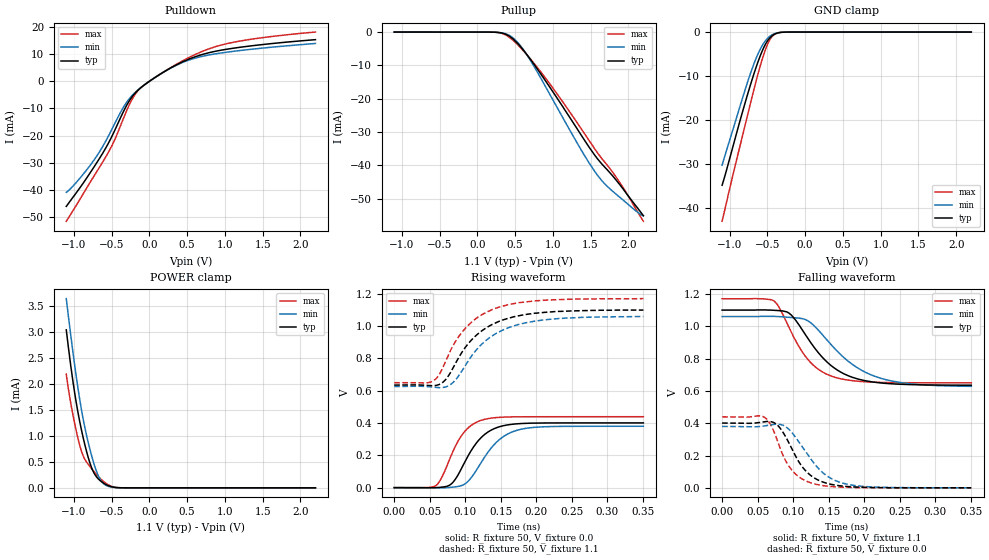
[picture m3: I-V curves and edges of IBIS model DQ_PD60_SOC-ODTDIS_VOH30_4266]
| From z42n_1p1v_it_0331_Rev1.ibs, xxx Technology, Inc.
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| DQ_PD60_SOC-ODTDIS_VOH30_4266
| (60 Ohm Pulldown, SOC ODT disabled setting, VOH=VDDQ/3.0 cal. point, 3200-4266Mbps)
[Model]   DQ_PD60_SOC-ODTDIS_VOH30_4266
Model_type   I/O
Vinl = 123.333mV
Vinh = 243.333mV
Vmeas = 183.333mV
Vref = 0.0mV
Cref = 0.0pF
|   typ   min   max
|C_comp   0.834pF   0.784pF   0.884pF
C_comp_pullup   0.4170pF   0.3920pF   0.4420pF
C_comp_pulldown   0.4170pF   0.3920pF   0.4420pF
| Note: C_comp changes when the ODT circuit is enabled.
[Model Spec]
| Input threshold voltage corners
Vinl   0.1233V   0.1167V   0.1350V
Vinh   0.2433V   0.2367V   0.2550V
| Measurement voltage corners
Vmeas   0.1833V   0.1767V   0.1950V
| Timing spec test load voltage corners
Vref   0.0000V   0.0000V   0.0000V
| Dynamic Overshoot Parameters from LPDDR4 Specification
D_overshoot_ampl_h   0.30   NA   NA
D_overshoot_ampl_l   0.30   NA   NA
D_overshoot_area_h   0.1n   NA   NA
D_overshoot_area_l   0.1n   NA   NA
[Voltage Range]   1.1000V   1.0600V   1.1700V
[Pullup Reference]   1.1000V   1.0600V   1.1700V
| Junction Temperature (Ambient temp is 35C typ 95C min -40C max)
[Temperature Range]   50.0   110.0   -40.0
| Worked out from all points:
|   slope of the pulldown table from 0 to 0.165 V, typ, clamps not added: 54.8 ohm
|   slope of the pullup table from 0 to 0.165 V, typ, clamps not added: 13 kohm
|   GND clamp passes 1 mA (typ) near -0.45 V on its own axis
|   POWER clamp passes 1 mA (typ) near -0.88 V on its own axis
|   rising waveform, R_fixture 50, V_fixture 0.0: 20-80 % time 35ps typ, 39ps min, 30.3ps max; typ from 0.001 V to 0.401 V
|   falling waveform, R_fixture 50, V_fixture 1.1: 20-80 % time 54ps typ, 66.1ps min, 43.5ps max; typ from 1.1 V to 0.635 V
|   rising waveform, R_fixture 50, V_fixture 1.1: 20-80 % time 55.1ps typ, 57.5ps min, 52.4ps max; typ from 0.635 V to 1.1 V
|   falling waveform, R_fixture 50, V_fixture 0.0: 20-80 % time 34.8ps typ, 42ps min, 30.2ps max; typ from 0.401 V to 0.001 V
[Pulldown]
|   Voltage   I(typ)   I(min)   I(max)
-1.1V     -46.14mA   -40.94mA   -51.62mA
-918.5mV  -39.24mA   -35.7mA    -43.49mA
-710.6mV  -30.65mA   -28.16mA   -33.97mA
-492.8mV  -20.14mA   -17.52mA   -23.58mA
-357.5mV  -12.02mA   -10.26mA   -14.71mA
-265.1mV  -7.208mA   -6.415mA   -8.684mA
-172.7mV  -3.892mA   -3.712mA   -4.234mA
-60.5mV   -1.24mA    -1.226mA   -1.224mA
411.4mV   6.776mA    6.592mA    7.095mA
893.2mV   11.15mA    10.18mA    12.89mA
1.365V    13.11mA    11.84mA    15.56mA
2.2V      15.34mA    13.95mA    18.15mA
[GND Clamp]
|   Voltage   I(typ)   I(min)   I(max)
-1.1V     -34.74mA   -30.21mA   -42.91mA
-1.047V   -31.66mA   -27.15mA   -39.02mA
-941.6mV  -25.02mA   -21.26mA   -31.32mA
-789.8mV  -15.72mA   -12.78mA   -20.72mA
-667.7mV  -8.907mA   -6.722mA   -12.29mA
-595.1mV  -5.399mA   -3.899mA   -7.688mA
-522.5mV  -2.666mA   -1.905mA   -3.811mA
-469.7mV  -1.359mA   -987.8uA   -1.786mA
-413.6mV  -563.7uA   -416.4uA   -619.9uA
-344.3mV  -144.1uA   -109.8uA   -124.4uA
-238.7mV  -9.035uA   -8.519uA   -5.04uA
2.2V      0A         0A         0A
[Pullup]
|   Voltage   I(typ)   I(min)   I(max)
-1.1V     6.275uA    9.671uA    2.829uA
229.9mV   -45.12uA   -45.81uA   -46.58uA
338.8mV   -360.2uA   -298.3uA   -496uA
434.5mV   -1.385mA   -1.132mA   -1.75mA
553.3mV   -3.878mA   -3.573mA   -4.208mA
691.9mV   -7.808mA   -8.045mA   -7.726mA
1.009V    -18.16mA   -20.62mA   -17.03mA
1.378V    -30.95mA   -35.41mA   -29.04mA
1.589V    -37.92mA   -42.84mA   -36.13mA
1.702V    -40.84mA   -45.82mA   -39.37mA
1.89V     -45.83mA   -49.59mA   -45.19mA
2.2V      -55.05mA   -55.17mA   -56.74mA
[POWER Clamp]
|   Voltage   I(typ)   I(min)   I(max)
-1.1V     3.033mA    3.633mA    2.184mA
-1.041V   2.345mA    2.929mA    1.625mA
-984.5mV  1.782mA    2.31mA     1.205mA
-911.9mV  1.201mA    1.61mA     764.7uA
-855.8mV  837.7uA    1.171mA    552.1uA
-779.9mV  447.9uA    701.4uA    396.3uA
-710.6mV  232.3uA    359.1uA    273.1uA
-657.8mV  146.8uA    178.8uA    190.7uA
-595.1mV  80.76uA    68.28uA    109.2uA
-482.9mV  15.73uA    9.557uA    19.51uA
-360.8mV  1.018uA    768.5nA    796.1nA
2.2V      0A         0A         0A
[Ramp]
|   typ   min   max
| 20% - 80%
dV/dt_r   240.24m/34.97p   227.79m/39.04p   263.30m/30.33p
dV/dt_f   278.79m/54.03p   259.05m/66.11p   312.07m/43.50p
| 25% - 75%
|dV/dt_r   200.20m/27.85p   189.82m/31.09p   219.41m/24.09p
|dV/dt_f   232.33m/43.03p   215.87m/52.69p   260.06m/34.62p
R_load = 50
[Rising Waveform]
R_fixture = 50
V_fixture = 0.0
|   Time   V(typ)   V(min)   V(max)
0s        701.6uV    613.5uV    508.4uV
58ps      514.8uV    -95.55uV   11.58mV
66ps      3.219mV    -535uV     55.51mV
78ps      15.84mV    1.701mV    175.5mV
87ps      58.39mV    5.992mV    264.1mV
99ps      155.2mV    21.91mV    346.3mV
125ps     320.7mV    173.6mV    420.4mV
150ps     379.7mV    304.4mV    436.1mV
179ps     397.3mV    362.2mV    439mV
351ps     401.1mV    380.3mV    439.3mV
[Falling Waveform]
R_fixture   = 50
V_fixture   = 1.1
V_fixture_min = 1.06
V_fixture_max = 1.17
|   Time   V(typ)   V(min)   V(max)
0s        1.1V       1.06V      1.17V
73ps      1.099V     1.061V     1.157V
94ps      1.082V     1.055V     995mV
118ps     943.4mV    1.04V      810mV
135ps     839.3mV    978.7mV    735.6mV
155ps     751.6mV    879mV      689.9mV
187ps     679.1mV    753.1mV    661.6mV
224ps     649mV      677.5mV    652.7mV
271ps     638.3mV    641.5mV    650.4mV
351ps     635.3mV    628.2mV    649.9mV
[Rising Waveform]
R_fixture   = 50
V_fixture   = 1.1
V_fixture_min = 1.06
V_fixture_max = 1.17
|   Time   V(typ)   V(min)   V(max)
0s        635mV      626.1mV    649.8mV
54ps      631.1mV    622.7mV    658.9mV
64ps      640mV      619.2mV    704.7mV
77ps      696.3mV    631.8mV    828.3mV
91ps      806.6mV    693.5mV    936mV
109ps     914.8mV    814.9mV    1.024V
127ps     981.8mV    902.8mV    1.079V
148ps     1.03V      965mV      1.118V
210ps     1.084V     1.038V     1.16V
351ps     1.099V     1.059V     1.17V
[Falling Waveform]
R_fixture = 50
V_fixture = 0.0
|   Time   V(typ)   V(min)   V(max)
0s        401.2mV    380.4mV    439.4mV
57ps      408mV      381.8mV    442.3mV
74ps      401.3mV    393.4mV    337.7mV
87ps      335.4mV    385.2mV    189.3mV
97ps      253.1mV    349.2mV    116.7mV
112ps     135.9mV    259.8mV    57.24mV
128ps     66.92mV    161.2mV    27.14mV
150ps     25.7mV     67.34mV    10.06mV
182ps     6.984mV    17.98mV    2.69mV
351ps     759.2uV    719uV      528.1uV
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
